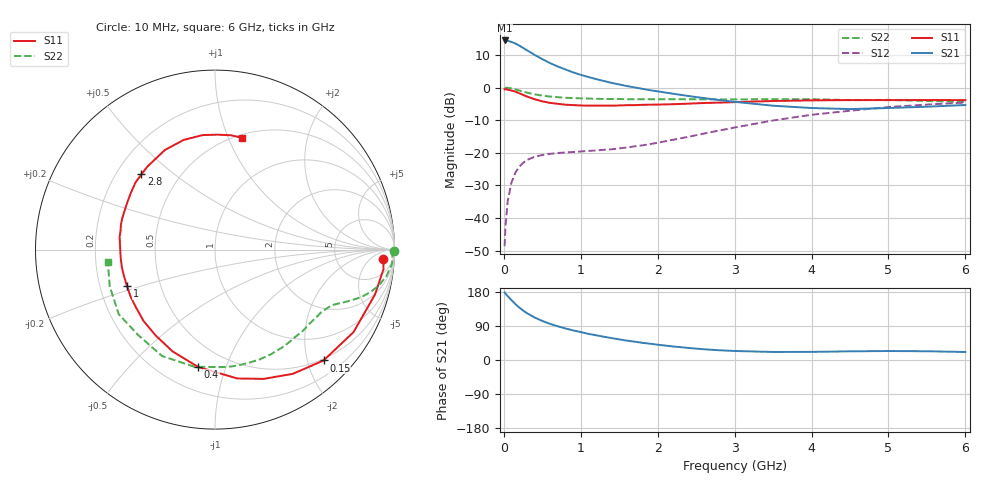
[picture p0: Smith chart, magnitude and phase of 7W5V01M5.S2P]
! Infineon Technologies  Discrete & RF Semiconductors
! BFS17W
! Si NPN RF Bipolar Junction Transistor in SOT323
! VCE = 5 V  IC = 1.5 mA
! Common Emitter S-Parameters:  August  1999
# GHz  S  MA  R  50
!  f  S11  S21  S12  S22
! GHz  MAG  ANG  MAG  ANG  MAG  ANG  MAG  ANG
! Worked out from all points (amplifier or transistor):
!   36 points, 10 MHz to 6 GHz, reference 50 ohm
!   highest |S21| = 14.4 dB at 10 MHz (marker M1)
!   |S21| within 3 dB of that: start of sweep to 300.6 MHz
!   unconditionally stable (mu >= 1): 922.6 MHz to 3.328 GHz; 3.986 GHz to end of sweep
!   at 250 MHz: K = 0.31, MSG = 17.6 dB, |S12| = -23.1 dB
!   at 1.4 GHz: K = 1.28, MAG = 7.0 dB, |S12| = -18.9 dB
!   at 6 GHz: K = 1.09, MAG = -2.2 dB, |S12| = -4.6 dB
!   S11 on the Smith chart (normalised r, x): 10 MHz: 18, -16; 150 MHz: 0.47, -2.30; 400 MHz: 0.35, -0.81; 1 GHz: 0.32, -0.18; 2.8 GHz: 0.30, +0.39; 6 GHz: 0.53, +1.12
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0.01  0.939 -3.1  5.262 178.4  0.0037 86.9  0.9999 -0.4
0.02  0.9452 -6.6  5.253 175.5  0.0071 91.4  0.9889 -1.8
0.05  0.9259 -15.7  5.203 168.5  0.018 81.4  0.9894 -4.6
0.1  0.8983 -30.8  4.997 157.9  0.0352 73.9  0.9667 -8.8
0.15  0.8646 -45.6  4.726 147.5  0.0496 65.1  0.934 -12.4
0.2  0.8165 -58.0  4.398 138.6  0.061 59.8  0.8993 -15.2
0.25  0.7694 -69.4  4.048 130.7  0.07 53.9  0.8649 -17.4
0.3  0.7286 -80.2  3.729 123.7  0.0775 50.0  0.8356 -19.1
0.4  0.6609 -98.1  3.166 112.1  0.0867 44.0  0.7859 -21.7
0.5  0.6145 -112.6  2.723 103.0  0.0923 40.3  0.7516 -23.5
0.6  0.5815 -124.7  2.368 95.4  0.0962 38.5  0.7268 -25.1
0.7  0.5627 -135.0  2.103 89.0  0.0991 37.9  0.7105 -26.8
0.8  0.5455 -143.8  1.89 83.3  0.1011 37.7  0.6976 -28.7
1  0.5306 -157.6  1.564 73.6  0.1045 39.2  0.6826 -32.3
1.1  0.528 -164.3  1.447 69.0  0.1067 40.6  0.6761 -34.6
1.6  0.5364 172.1  1.052 51.1  0.1204 50.5  0.6618 -46.2
2.2  0.5549 151.7  0.803 35.7  0.1581 62.1  0.661 -62.1
2.8  0.5868 134.4  0.642 25.7  0.2191 66.5  0.6582 -79.3
3.5  0.6212 116.7  0.526 21.2  0.3125 64.2  0.6628 -99.9
4.5  0.6417 96.2  0.467 22.9  0.4403 52.2  0.6404 -131.9
5.5  0.6431 82.0  0.508 23.1  0.5476 38.8  0.6214 -160.7
6  0.6409 76.6  0.539 21.1  0.5884 32.5  0.601 -173.4
